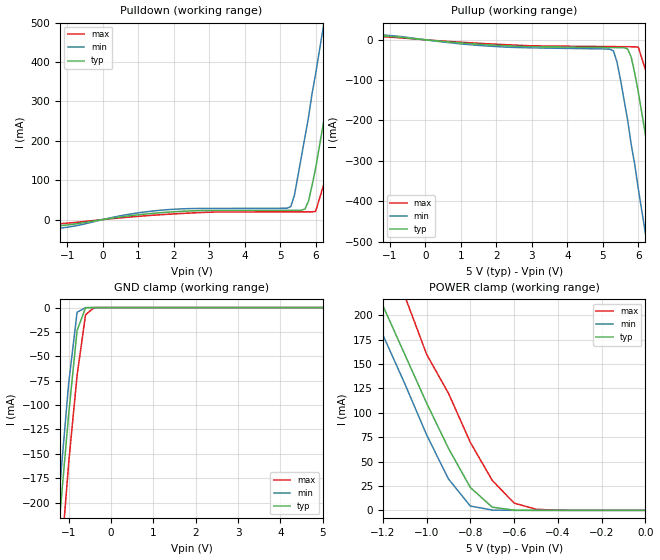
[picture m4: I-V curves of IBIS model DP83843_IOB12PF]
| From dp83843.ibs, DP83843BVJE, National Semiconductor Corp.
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|   Model IOB12PF
[Model]   DP83843_IOB12PF
Model_type   I/O
Polarity   Non-Inverting
Enable   Active-High
Vinl =   0.80V
Vinh =   2.00V
Vmeas =   1.50V
Cref =  10.00pF
Rref =  50.00
C_comp   5.83pF   5.83pF   5.83pF
[Temperature Range]   50.00   -15.00   0.15k
[Voltage Range]   5.00V   4.50V   5.50V
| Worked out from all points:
|   slope of the pulldown table from 0 to 0.75 V, typ, clamps not added: 79.1 ohm
|   slope of the pullup table from 0 to 0.75 V, typ, clamps not added: 124 ohm
|   GND clamp passes 1 mA (typ) near -0.61 V on its own axis
|   POWER clamp passes 1 mA (typ) near -0.63 V on its own axis
[Pulldown]
| voltage   I(typ)   I(min)   I(max)
-5V       -34.8mA    -35.6mA    -35.88mA
-1.8V     -20.78mA   -28.15mA   -14.54mA
1.9V      19.16mA    25.54mA    13.78mA
5.2V      23.43mA    28.97mA    19.51mA
5.4V      23.45mA    60.81mA    19.53mA
5.7V      26.74mA    210mA      19.56mA
5.8V      46.88mA    260mA      19.57mA
6V        130mA      370mA      20.72mA
6.4V      340mA      590mA      140mA
6.8V      560mA      820mA      340mA
7.2V      790mA      1.04A      560mA
10V       2.36A      2.63A      2.12A
[Pullup]
| voltage   I(typ)   I(min)   I(max)
-5V       19.56mA    17.24mA    23.39mA
-1.8V     12.71mA    15.07mA    10.47mA
5.2V      -19.16mA   -23.39mA   -16.8mA
5.3V      -19.25mA   -27.77mA   -16.86mA
5.4V      -19.34mA   -55.76mA   -16.93mA
5.7V      -22.93mA   -200mA     -17.14mA
5.8V      -43.2mA    -260mA     -17.21mA
6V        -130mA     -370mA     -18.42mA
6.4V      -340mA     -590mA     -130mA
6.8V      -560mA     -820mA     -340mA
7.2V      -780mA     -1.04A     -550mA
10V       -2.37A     -2.64A     -2.12A
[GND_clamp]
| voltage   I(typ)   I(min)   I(max)
-5V       -2.34A     -2.33A     -2.38A
-1.4V     -320mA     -290mA     -370mA
-1.2V     -210mA     -180mA     -270mA
-1V       -110mA     -78.16mA   -160mA
-800mV    -23.51mA   -4.82mA    -69.47mA
-600mV    -200uA     -68.15uA   -7.33mA
-400mV    -240nA     -54.77nA   -97.41uA
5V        37.44pA    220nA      -290pA
[POWER_clamp]
| voltage   I(typ)   I(min)   I(max)
-5V       2.34A      2.31A      2.38A
-1.3V     270mA      230mA      320mA
-1.2V     210mA      180mA      270mA
-1.1V     160mA      130mA      220mA
-1V       110mA      77.42mA    160mA
-900mV    63.54mA    32.11mA    120mA
-800mV    23.39mA    4.41mA     69.55mA
-700mV    3.26mA     300uA      30.7mA
-600mV    220uA      7.78uA     7.44mA
-500mV    7.36uA     220nA      1.14mA
-400mV    210nA      6.2nA      110uA
0V        37.44pA    31.64pA    1.91nA
[Ramp]
| variable   typ   min   max
dV/dt_r   0.54/0.86n   0.62/0.58n   0.49/1.27n
dV/dt_f   0.70/0.58n   0.85/0.41n   0.58/0.81n
R_load = 50.00
|[Rising Waveform]
|R_fixture = 0.50k
|V_fixture = 0.000
| Note: If your simulator can handle R_fixture = 0.5k then you
|   can un-comment the Rising and Falling Waveform sections
| time   V(typ)   V(min)   V(max)
|  0.000S   -17.58uV   69.47uV   -28.04uV
|   0.40nS   -17.83mV   29.38mV   -1.50mV
|   0.80nS   0.18V   0.62V   -20.46mV
|   1.20nS   0.85V   2.37V   0.21V
|   1.60nS   2.26V   3.47V   0.75V
|   2.00nS   3.15V   3.74V   1.68V
|   2.40nS   3.82V   3.78V   2.62V
|   2.80nS   3.94V   3.78V   3.30V
|   3.20nS   3.97V   3.78V   3.82V
|   3.60nS   3.98V   3.78V   4.01V
|   4.00nS   3.98V   3.78V   4.06V
|   4.40nS   3.98V   3.78V   4.08V
|   4.80nS   3.98V   3.78V   4.08V
|   5.20nS   3.98V   3.78V   4.08V
|   5.60nS   3.98V   3.78V   4.08V
|   6.00nS   3.98V   3.78V   4.08V
|   6.40nS   3.98V   3.78V   4.08V
|   6.80nS   3.98V   3.78V   4.08V
|   7.20nS   3.98V   3.78V   4.08V
|   7.60nS   3.98V   3.78V   4.08V
|   8.00nS   3.98V   3.78V   4.08V
|   8.40nS   3.98V   3.78V   4.08V
|   8.80nS   3.98V   3.78V   4.08V
|   9.20nS   3.98V   3.78V   4.08V
|   9.60nS   3.98V   3.78V   4.08V
|  10.00nS   3.98V   3.78V   4.08V
|  10.40nS   3.98V   3.78V   4.08V
|  10.80nS   3.98V   3.78V   4.08V
|  11.20nS   3.98V   3.78V   4.08V
|  11.60nS   3.98V   3.78V   4.08V
|  12.00nS   3.98V   3.78V   4.08V
|  12.40nS   3.98V   3.78V   4.08V
|  12.80nS   3.98V   3.78V   4.08V
|  13.20nS   3.98V   3.78V   4.08V
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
